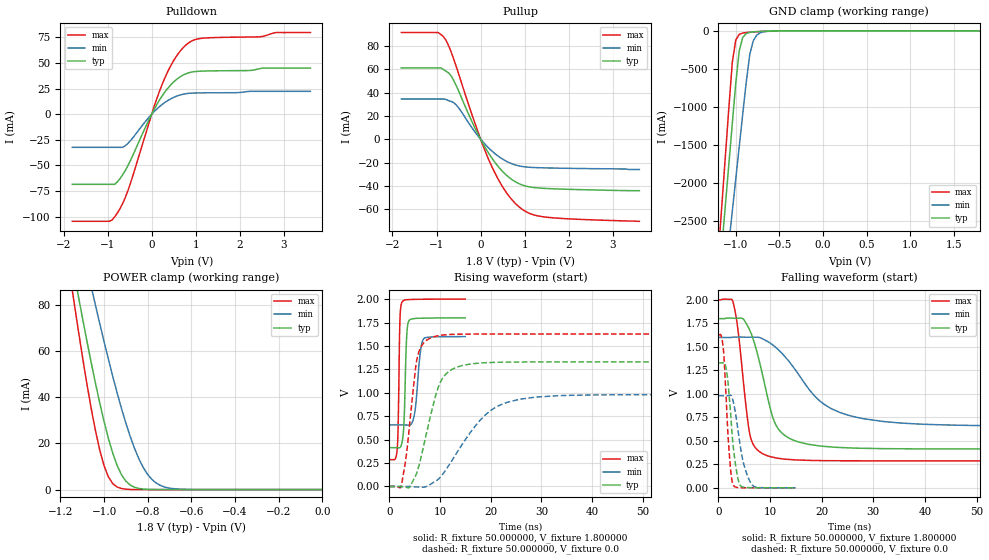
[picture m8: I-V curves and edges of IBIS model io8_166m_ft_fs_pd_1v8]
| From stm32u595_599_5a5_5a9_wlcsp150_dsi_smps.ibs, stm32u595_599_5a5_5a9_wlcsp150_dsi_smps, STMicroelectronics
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|   Model io8_166m_ft_fs_pd_1v8
[Model]  io8_166m_ft_fs_pd_1v8
Model_type I/O
Polarity   Non-Inverting
Enable   Active-Low
Vinl =   0.540000V
Vinh =   1.260000V
Vmeas =  0.900000V
Cref =   50.000000pF
Rref =   100.000000M
Vref =   0.0V
C_comp   3.358200pF   3.352700pF   3.400300pF
[Temperature Range]   25.000000   0.140000k   -40.000000
[Pullup Reference]   1.800000V   1.600000V   2.000000V
[Pulldown Reference]   0.0V   0.0V   0.0V
[POWER Clamp Reference]   1.800000V   1.600000V   2.000000V
[GND Clamp Reference]   0.0V   0.0V   0.0V
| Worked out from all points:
|   slope of the pulldown table from 0 to 0.27 V, typ, clamps not added: 13.6 ohm
|   slope of the pullup table from 0 to 0.27 V, typ, clamps not added: 15.9 ohm
|   GND clamp passes 1 mA (typ) near -0.50 V on its own axis
|   POWER clamp passes 1 mA (typ) near -0.86 V on its own axis
|   rising waveform, R_fixture 50.000000, V_fixture 1.800000: 20-80 % time 455ps typ, 905ps min, 302ps max; typ from 0.414 V to 1.8 V
|   rising waveform, R_fixture 50.000000, V_fixture 0.0: 20-80 % time 3.64ns typ, 7.99ns min, 1.94ns max; typ from 0 V to 1.33 V
|   falling waveform, R_fixture 50.000000, V_fixture 1.800000: 20-80 % time 3.88ns typ, 9.14ns min, 2.06ns max; typ from 1.8 V to 0.414 V
|   falling waveform, R_fixture 50.000000, V_fixture 0.0: 20-80 % time 1.31ns typ, 1.87ns min, 980ps max; typ from 1.33 V to 0 V
[Pulldown]
|Voltage   I(typ)   I(min)   I(max)
-1.8V     -68.38mA   -32.32mA   -104.4mA
-960mV    -68.38mA   -32.32mA   -104.4mA
-780mV    -66.08mA   -32.32mA   -96.43mA
-660mV    -59.2mA    -32.31mA   -87.22mA
-540mV    -50.22mA   -28.51mA   -74.66mA
0V        -10fA      -200fA     0A
240mV     18.04mA    9.6mA      29.42mA
480mV     30.68mA    16.02mA    50.95mA
780mV     39.48mA    19.99mA    67.56mA
1.14V     41.99mA    20.78mA    74.01mA
2.82V     44.93mA    22.28mA    79.57mA
3.6V      44.93mA    22.28mA    79.57mA
[Pullup]
|Voltage   I(typ)   I(min)   I(max)
-1.8V     61.23mA    34.57mA    91.65mA
-960mV    61.23mA    34.57mA    91.65mA
-840mV    59.79mA    34.57mA    88.02mA
-720mV    56.82mA    33.03mA    79.77mA
-600mV    49.68mA    31.11mA    67.64mA
-120mV    9.014mA    5.781mA    12.75mA
240mV     -15.38mA   -9.6mA     -22.37mA
540mV     -29.31mA   -18.02mA   -43.36mA
900mV     -38.69mA   -23.13mA   -58.99mA
1.14V     -41.14mA   -24.16mA   -64.17mA
1.5V      -42.31mA   -24.64mA   -67mA
3.6V      -44.2mA    -26mA      -70.5mA
[GND_clamp]
|Voltage   I(typ)   I(min)   I(max)
-1.8V     -9.908A    -9.683A    -9.994A
-1.2V     -3.383A    -4.084A    -2.934A
-1.16V    -2.841A    -3.655A    -2.294A
-1.12V    -2.299A    -3.226A    -1.656A
-1.04V    -1.218A    -2.369A    -414.2mA
-1V       -684.7mA   -1.941A    -119.2mA
-960mV    -257.2mA   -1.514A    -45.67mA
-920mV    -87.04mA   -1.089A    -28.94mA
-840mV    -19.36mA   -312.8mA   -18.98mA
-800mV    -13.56mA   -132.4mA   -15.51mA
-720mV    -8.053mA   -25.67mA   -9.505mA
1.8V      45.71uA    33.32uA    56.11uA
[POWER_clamp]
|Voltage   I(typ)   I(min)   I(max)
-1.8V     470.8mA    433.7mA    554.6mA
-1.14V    95.25mA    122.7mA    82.82mA
-1.12V    84.97mA    114mA      70.27mA
-1.06V    55.51mA    88.42mA    35.67mA
-1.04V    46.34mA    80.15mA    25.76mA
-1V       29.51mA    64.13mA    10.3mA
-940mV    10.39mA    41.86mA    1.109mA
-900mV    3.624mA    28.77mA    182.8uA
-840mV    490.7uA    13.24mA    11.35uA
-800mV    116.8uA    6.532mA    1.77uA
-740mV    13.2uA     1.724mA    109.3nA
0V        0A         18.75nA    0A
[Ramp]
| variable   typ   min   max
dV/dt_r  0.79740/3.63428n   0.58783/7.98171n   0.97632/1.93010n
dV/dt_f  0.83143/3.86975n   0.56586/9.13286n   1.02744/2.05024n
R_load = 50.000000
[Rising Waveform]
R_fixture= 50.000000
V_fixture= 1.800000
V_fixture_min= 1.600000
V_fixture_max= 2.000000
|time   V(typ)   V(min)   V(max)
0s        413.8mV    656.4mV    287.1mV
1.592ns   413.2mV    656.4mV    435mV
2.072ns   414.9mV    656.4mV    1.763V
2.462ns   463.7mV    656.4mV    1.965V
2.883ns   685.1mV    656.3mV    1.987V
3.423ns   1.612V     655.4mV    1.994V
3.844ns   1.768V     654mV      1.994V
5.045ns   1.793V     803.1mV    1.997V
6.637ns   1.796V     1.566V     1.998V
14.95ns   1.8V       1.599V     2V
[Rising Waveform]
R_fixture= 50.000000
V_fixture= 0.0
V_fixture_min= 0.0
V_fixture_max= 0.0
|time   V(typ)   V(min)   V(max)
0s        2.606uV    2.596uV    1.309uV
2.402ns   -3.718mV   1.088uV    20.59mV
3.403ns   -10.83mV   105.5uV    358.7mV
5.005ns   96.78mV    -4.369mV   1.188V
6.206ns   303mV      -6.927mV   1.487V
9.209ns   985.4mV    59.75mV    1.605V
13.21ns   1.271V     352.1mV    1.624V
19.22ns   1.321V     777.7mV    1.627V
25.83ns   1.328V     931.9mV    1.627V
99.7ns    1.329V     979.8mV    1.627V
[Falling Waveform]
R_fixture= 50.000000
V_fixture= 1.800000
V_fixture_min= 1.600000
V_fixture_max= 2.000000
|time   V(typ)   V(min)   V(max)
0s        1.8V       1.599V     2V
2.803ns   1.805V     1.603V     1.986V
3.804ns   1.804V     1.604V     1.679V
6.206ns   1.66V      1.602V     542.8mV
9.61ns    944.3mV    1.554V     339mV
11.21ns   662mV      1.49V      317.5mV
13.61ns   531.3mV    1.349V     302.5mV
19.82ns   444.2mV    916.4mV    289.9mV
28.03ns   420.8mV    735.7mV    287.5mV
99.7ns    413.8mV    656.4mV    287.1mV
[Falling Waveform]
R_fixture= 50.000000
V_fixture= 0.0
V_fixture_min= 0.0
V_fixture_max= 0.0
|time   V(typ)   V(min)   V(max)
0s        1.329V     979.8mV    1.627V
510.5ps   1.329V     979.8mV    1.623V
961ps     1.332V     979.8mV    1.485V
1.562ns   1.255V     979.6mV    908.1mV
2.252ns   879.4mV    986.2mV    271.7mV
2.883ns   440.1mV    916.9mV    31.34mV
4.114ns   38.78mV    494.1mV    2.566mV
4.985ns   6.551mV    239mV      1.293mV
6.547ns   1.958mV    31.77mV    597.3uV
14.95ns   2.606uV    2.596uV    1.309uV
